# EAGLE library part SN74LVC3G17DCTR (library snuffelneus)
TRIPLE SCHMITT-TRIGGER BUFFER
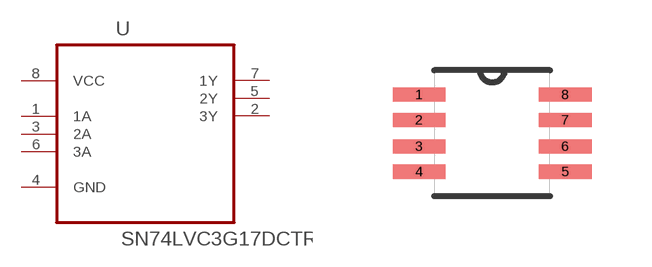
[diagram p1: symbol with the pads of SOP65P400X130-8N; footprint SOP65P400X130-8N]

Designator prefix U

## SN74LVC3G17DCTR (MPN: SN74LVC3G17DCTR; OC_FARNELL: 1236391; OC_NEWARK: 90H3713; PACKAGE: SSOP-8; SUPPLIER: Texas Instruments)  [SOP65P400X130-8N]
1  1A  in
2  3Y  out
3  2A  in
4  GND  pas
5  2Y  out
6  3A  in
7  1Y  out
8  VCC  pwr

## Footprint SOP65P400X130-8N (pad centres in mm)
smd 1.321 x 0.356: 1 -1.829,0.965; 2 -1.829,0.33; 3 -1.829,-0.33; 4 -1.829,-0.965; 5 1.829,-0.965; 6 1.829,-0.33; 7 1.829,0.33; 8 1.829,0.965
